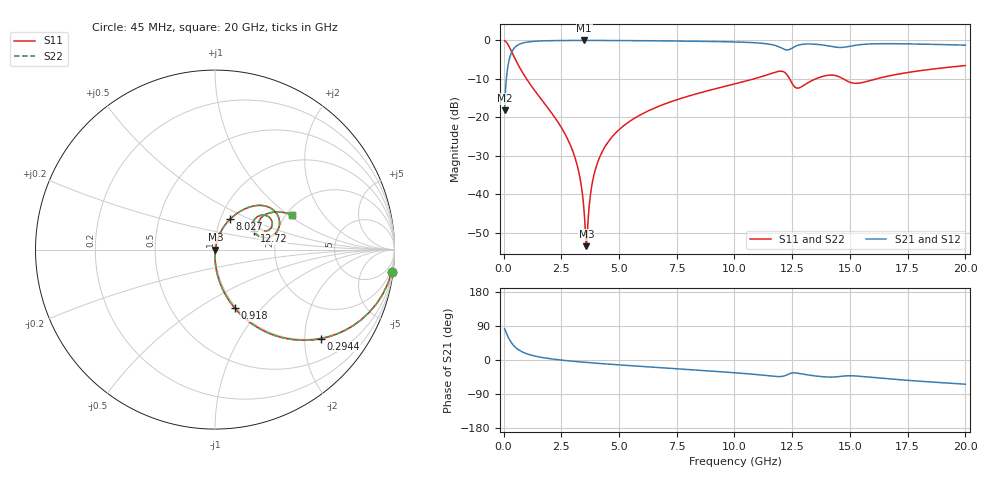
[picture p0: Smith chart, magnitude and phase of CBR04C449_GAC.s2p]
! S-parameter model data by Modelithics Inc.  support@modelithics.com 813-866-6335  Tampa FL USA
! S-Parameter data specifications:
! Substrate: 20-mil Rogers 4350B, substrate thickness, H=0.508mm, Dielectric constant, Er=3.75
! PCB Mounting Pad Footprint: Pad width, PadW=0.52mm , Pad length, PadL=0.52mm , Pad gap, PadG (edge-to-edge)=0.28mm , Reference planes=1.32mm apart
#  GHz  S  MA  R 50
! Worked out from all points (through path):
!   801 points, 45 MHz to 20 GHz, reference 50 ohm
!   highest |S21| = -0.02 dB at 3.487 GHz (marker M1); lowest = -18.1 dB at 45 MHz (marker M2)
!   group delay of S21, straight-line fit = 11.1 ps
!   lowest |S11| = -53.4 dB at 3.587 GHz (marker M3), VSWR 1.00, Z = 50.2 - j0.0223 ohm
!   |S11| at or under -10 dB: 994.7 MHz to 10.84 GHz (9.841 GHz wide, 166 % of centre); 12.39 GHz to 13.51 GHz (1.121 GHz wide, 8.66 % of centre); 14.71 GHz to 16.14 GHz (1.426 GHz wide, 9.25 % of centre)
!   |S22| runs from -53.4 to -0.1 dB; largest |S21 - S12| = 0
!   S11 on the Smith chart (normalised r, x): 45 MHz: 1, -16; 294.4 MHz: 0.98, -2.40; 918 MHz: 0.98, -0.72; 8.027 GHz: 1.11, +0.39; 12.72 GHz: 1.51, +0.33; 20 GHz: 2.14, +1.07
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0.045  0.9922 -7.2  0.1243 82.8  0.1243 82.8  0.9922 -7.2
0.194662  0.8785 -28.9  0.4774 61.1  0.4774 61.1  0.8785 -28.9
0.294438  0.7711 -40.0  0.6362 49.9  0.6362 49.9  0.7711 -40.0
0.568819  0.5241 -59.3  0.8509 30.6  0.8509 30.6  0.5241 -59.3
0.918031  0.3434 -71.4  0.9381 18.4  0.9381 18.4  0.3434 -71.4
2.738925  0.05494 -89.8  0.9965 -1.7  0.9965 -1.7  0.05494 -89.8
3.138025  0.02713 -89.8  0.9975 -4.1  0.9975 -4.1  0.02713 -89.8
3.387462  0.01175 -85.2  0.9978 -5.4  0.9978 -5.4  0.01175 -85.2
3.487237  0.00607 -75.6  0.9978 -5.9  0.9978 -5.9  0.00607 -75.6
3.587013  0.002132 -6.0  0.9978 -6.4  0.9978 -6.4  0.002132 -6.0
3.911281  0.01775 74.8  0.9975 -8.0  0.9975 -8.0  0.01775 74.8
4.385212  0.04129 76.5  0.9966 -10.2  0.9966 -10.2  0.04129 76.5
5.283188  0.08148 74.0  0.9939 -14.1  0.9939 -14.1  0.08148 74.0
6.704981  0.1388 68.8  0.987 -19.9  0.987 -19.9  0.1388 68.8
8.027  0.1898 63.6  0.9776 -25.3  0.9776 -25.3  0.1898 63.6
10.0225  0.273 54.6  0.9538 -33.7  0.9538 -33.7  0.273 54.6
12.018  0.398 28.2  0.8013 -43.6  0.8013 -43.6  0.398 28.2
12.71642  0.24 25.2  0.8571 -34.6  0.8571 -34.6  0.24 25.2
13.36496  0.3018 37.7  0.8959 -41.0  0.8959 -41.0  0.3018 37.7
14.86159  0.2987 20.3  0.8242 -41.8  0.8242 -41.8  0.2987 20.3
16.68248  0.3453 34.8  0.9062 -49.9  0.9062 -49.9  0.3453 34.8
20  0.4713 24.4  0.8676 -63.9  0.8676 -63.9  0.4713 24.4
